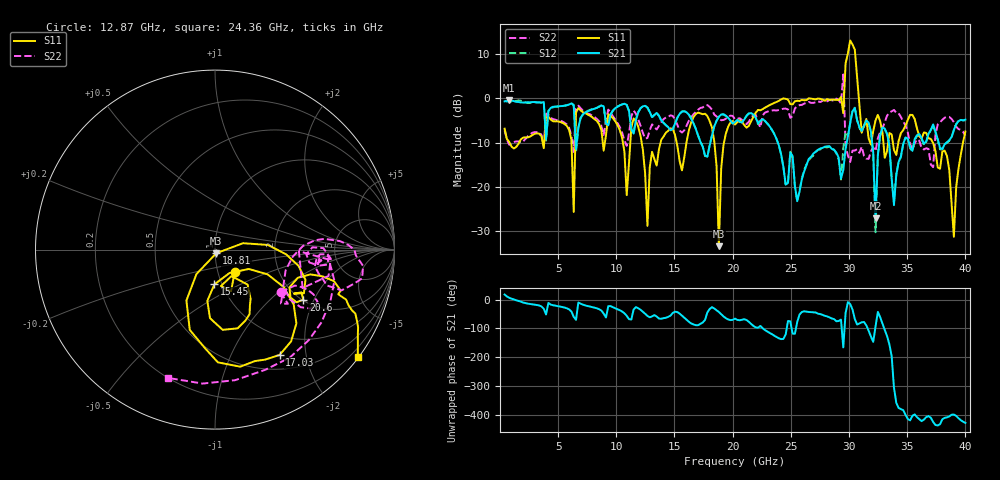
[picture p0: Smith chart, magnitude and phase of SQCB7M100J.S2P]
! Network Analyzer HP8722ES.07.66: Jul 25, 2000 Serial No. US39175408
! 26 Oct 2004  16:03:59
! Frequency  S11  S21  S12  S22
# HZ  S  DB R  50
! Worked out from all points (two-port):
!   201 points, 400 MHz to 40 GHz, reference 50 ohm
!   highest |S21| = -0.42 dB at 796 MHz (marker M1); lowest = -27.1 dB at 32.28 GHz (marker M2)
!   |S21| within 3 dB of the highest: start of sweep to 3.827 GHz; 4.146 GHz to 6.377 GHz (2.231 GHz wide, 42.4 % of centre)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
!   lowest |S11| = -33.4 dB at 18.81 GHz (marker M3), VSWR 1.04, Z = 50.7 - j2.05 ohm
!   |S11| at or under -10 dB: 823.2 MHz to 1.651 GHz (827.5 MHz wide, 66.9 % of centre); 12.18 GHz to 13.81 GHz (1.628 GHz wide, 12.5 % of centre); 37.2 GHz to 39.8 GHz (2.595 GHz wide, 6.74 % of centre)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
!   |S22| runs from -15.6 to 5.4 dB; largest |S21 - S12| = 0.15
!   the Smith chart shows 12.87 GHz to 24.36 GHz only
!   S11 on the Smith chart (normalised r, x): 12.87 GHz: 1.20, -0.31; 15.45 GHz: 0.92, -0.37; 17.03 GHz: 0.70, -1.56; 18.81 GHz: 1.01, -0.04; 20.6 GHz: 2.02, -1.66; 24.36 GHz: 0.03, -3.00
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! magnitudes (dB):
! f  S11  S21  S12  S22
! 400 MHz  -6.9  -0.7  -0.6  -7.3
! 796 MHz  -9.9  -0.4  -0.8  -10.5
! 5.746 GHz  -6.2  -1.6  -1.6  -5.9
! 6.34 GHz  -25.7  -1.6  -1.6  -12.1
! 7.132 GHz  -3.2  -3.6  -3.7  -2.8
! 12.87 GHz  -15.6  -3.1  -3.2  -7.2
! 13.67 GHz  -11.5  -3.9  -4.0  -6.2
! 15.45 GHz  -14.3  -3.5  -3.5  -7.3
! 17.03 GHz  -3.2  -8.5  -8.4  -2.6
! 18.42 GHz  -9.8  -6.4  -6.2  -3.7
! 18.81 GHz  -33.4  -4.2  -4.2  -4.5
! 20.2 GHz  -6.0  -5.4  -5.3  -4.8
! 20.6 GHz  -5.0  -5.3  -5.4  -4.5
! 24.36 GHz  -0.1  -15.5  -15.6  -2.4
! 26.93 GHz  -0.2  -12.5  -12.9  -1.1
! 29.51 GHz  -3.4  -16.2  -11.2  5.4
! 30.1 GHz  13.0  -5.6  -5.6  -14.4
! 31.68 GHz  -9.1  -5.5  -5.6  -13.7
! 32.28 GHz  -5.0  -27.1  -30.3  -11.9
! 33.47 GHz  -7.9  -10.7  -11.0  -3.3
! 39.01 GHz  -31.3  -7.2  -7.2  -5.4
! 40 GHz  -7.5  -4.8  -5.0  -8.5
